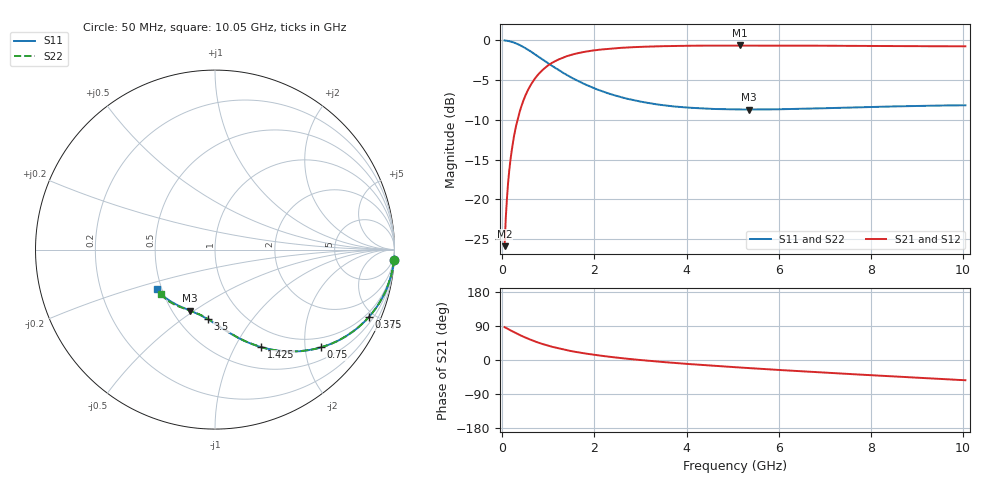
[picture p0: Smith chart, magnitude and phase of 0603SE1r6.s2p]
! AVX Thin Film Operation		Date: August 2001
! Description: Accu-P® Series, Thin Film, SMD, RF Capacitor
! Part Number: 06035J1R6ABT
! 50 MHz  -  10.05 GHz
! Serial Measurements
# mhz S db R 50
!	S11		S21		S12		S22
!	dB	Phase	dB	Phase	dB	Phase	dB	Phase
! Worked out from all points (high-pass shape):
!   401 points, 50 MHz to 10.05 GHz, reference 50 ohm
!   highest |S21| = -0.64 dB at 5.15 GHz (marker M1); lowest = -25.9 dB at 50 MHz (marker M2)
!   |S21| within 3 dB of the highest: 890.2 MHz to end of sweep
!   lowest |S11| = -8.7 dB at 5.35 GHz (marker M3), VSWR 2.16, Z = 30.6 - j24.1 ohm
!   |S11| at or under -10 dB: nowhere
!   |S22| runs from -8.7 to 0.0 dB; largest |S21 - S12| = 0
!   S11 on the Smith chart (normalised r, x): 50 MHz: 1, -35; 375 MHz: 0.77, -4.63; 750 MHz: 0.77, -2.34; 1.425 GHz: 0.75, -1.28; 3.5 GHz: 0.69, -0.63; 10.05 GHz: 0.47, -0.25
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50  -0.01 -3.3  -25.90 86.7  -25.90 86.7  -0.01 -3.3
75  -0.03 -5.0  -22.41 85.0  -22.41 85.0  -0.03 -5.0
125  -0.07 -8.3  -17.98 81.7  -17.98 81.7  -0.07 -8.3
150  -0.10 -9.8  -16.43 80.2  -16.43 80.2  -0.10 -9.8
200  -0.17 -13.1  -14.04 76.9  -14.04 76.9  -0.17 -13.1
275  -0.32 -17.7  -11.43 72.3  -11.43 72.3  -0.32 -17.7
375  -0.58 -23.8  -9.04 66.2  -9.04 66.2  -0.58 -23.8
550  -1.15 -33.3  -6.33 56.7  -6.33 56.7  -1.15 -33.3
750  -1.91 -42.7  -4.49 47.2  -4.49 47.2  -1.91 -42.7
1050  -3.08 -54.0  -2.95 36.0  -2.95 36.0  -3.08 -54.0
1425  -4.43 -64.8  -1.95 25.2  -1.95 25.2  -4.43 -64.7
1725  -5.33 -71.3  -1.51 18.7  -1.51 18.7  -5.33 -71.2
2075  -6.21 -77.7  -1.19 12.3  -1.19 12.3  -6.21 -77.5
2450  -6.94 -83.4  -0.99 6.7  -0.99 6.7  -6.94 -83.0
3400  -8.09 -94.7  -0.74 -4.5  -0.74 -4.5  -8.08 -93.9
3500  -8.17 -95.7  -0.73 -5.5  -0.73 -5.5  -8.16 -94.9
5050  -8.69 -110.0  -0.65 -19.0  -0.65 -19.0  -8.68 -108.0
5150  -8.70 -110.7  -0.65 -19.8  -0.65 -19.8  -8.68 -108.7
5350  -8.70 -112.1  -0.65 -21.3  -0.65 -21.3  -8.69 -110.1
6725  -8.58 -122.0  -0.67 -31.3  -0.67 -31.3  -8.56 -120.0
8400  -8.33 -134.2  -0.71 -42.8  -0.71 -42.8  -8.30 -130.2
10050  -8.17 -145.6  -0.75 -53.3  -0.75 -53.3  -8.14 -140.6
